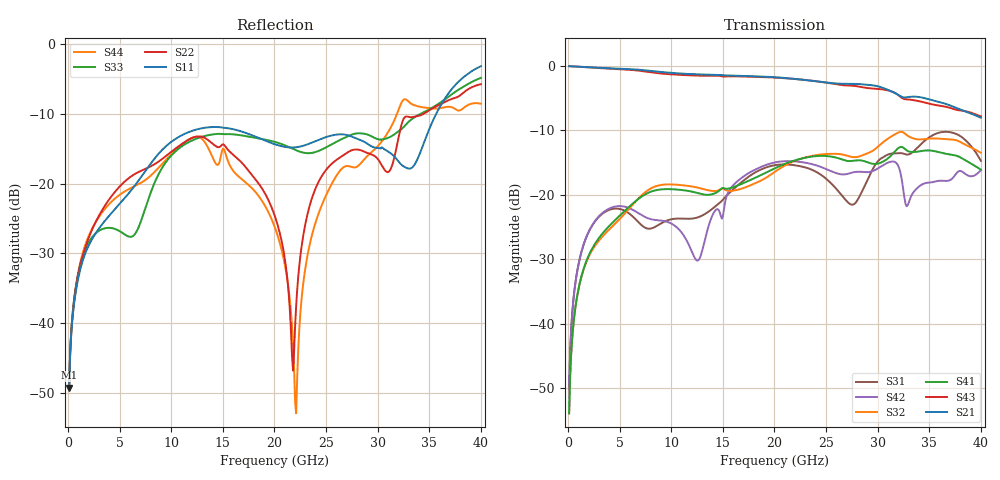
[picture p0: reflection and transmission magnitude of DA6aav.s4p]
! ADC12DJ2700AAV, ADC12DJ3200AAV, ADC08DJ3200AAV
! 144 pin AAV package
! Texas Instruments 4/21/2021
! Single-ended  S-parameters
! PORT#  PORT_NAME  NET_NAME
! PORT1:  DAxN.DIEBUMP DAxN
! PORT2:  DAxN.BGA  DAxN
! PORT3:  DAxP.DIEBUMP DAxP
! PORT4:  DAxP.BGA  DAxP
! Touchstone Ver. 1.0
! Number of ports is 4
# Hz	S	MA	R	50.000000
! SCATTERING PARAMETERS  :
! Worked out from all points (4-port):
!   400 points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, 100 MHz to 40 GHz, reference 50 ohm
!   strongest paths, dB at 100 MHz, 10.1 GHz, 20.1 GHz, 30.1 GHz, 40 GHz:
!     S21: 0.0, -1.1, -1.7, -3.2, -8.0
!     S43: 0.0, -1.3, -1.8, -3.5, -7.8
!     S41: -53.9, -19.1, -15.8, -15.1, -16.1
!     S32: -53.9, -18.4, -16.3, -12.4, -13.5
!     S42: -50.2, -24.5, -14.9, -15.8, -16.1
!     S31: -50.2, -23.7, -15.4, -14.6, -14.7
!   lowest |S11| = -49.3 dB at 100 MHz (marker M1), VSWR 1.01, Z = 50.2 + j0.295 ohm
!   |S11| at or under -10 dB: start of sweep to 35.66 GHz
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1e8  0.003426 58.9  0.998 -1.4  0.003104 84.8  0.002018 -97.1
     0.998 -1.4  0.003443 57.8  0.002018 -97.1  0.003101 84.6
     0.003104 84.8  0.002018 -97.1  0.003439 62.0  0.9981 -1.3
     0.002018 -97.1  0.003101 84.6  0.9981 -1.3  0.003442 61.3
2.8e9  0.04545 56.0  0.972 -36.3  0.06509 46.8  0.04405 -144.3
       0.972 -36.3  0.05535 12.4  0.0423 -142.9  0.06561 40.4
       0.06509 46.8  0.0423 -142.9  0.04479 41.7  0.9676 -34.1
       0.04405 -144.3  0.06561 40.4  0.9676 -34.1  0.05482 18.0
1.46e10  0.2545 -25.7  0.8539 179.0  0.08566 56.7  0.1073 58.5
         0.8539 179.0  0.1825 -135.3  0.1088 63.6  0.07631 80.6
         0.08566 56.7  0.1088 63.6  0.2276 -5.2  0.8407 -166.8
         0.1073 58.5  0.07631 80.6  0.8407 -166.8  0.1384 -126.0
2.03e10  0.1889 -58.4  0.8168 108.0  0.1713 33.6  0.1646 -6.4
         0.8168 108.0  0.05062 -178.2  0.1561 15.5  0.1803 -3.0
         0.1713 33.6  0.1561 15.5  0.1967 -48.5  0.8122 127.8
         0.1646 -6.4  0.1803 -3.0  0.8122 127.8  0.0425 -172.3
2.21e10  0.1824 -58.0  0.7928 84.9  0.1692 21.9  0.1866 -33.6
         0.7928 84.9  0.01327 -39.3  0.1855 -9.7  0.1816 -32.9
         0.1692 21.9  0.1855 -9.7  0.1736 -56.6  0.7924 106.3
         0.1866 -33.6  0.1816 -32.9  0.7924 106.3  0.002246 -73.7
2.59e10  0.2243 -71.4  0.7336 37.5  0.1135 8.1  0.1954 -95.3
         0.7336 37.5  0.1461 -67.9  0.2085 -65.7  0.1484 -113.7
         0.1135 8.1  0.2085 -65.7  0.1978 -64.1  0.7241 60.9
         0.1954 -95.3  0.1484 -113.7  0.7241 60.9  0.1107 -36.0
4e10  0.6968 -37.1  0.3971 -146.8  0.1837 -45.9  0.1569 43.5
      0.3971 -146.8  0.5175 -103.9  0.2122 70.3  0.1558 69.0
      0.1837 -45.9  0.2122 70.3  0.5742 49.0  0.4074 -101.2
      0.1569 43.5  0.1558 69.0  0.4074 -101.2  0.3746 -107.4
